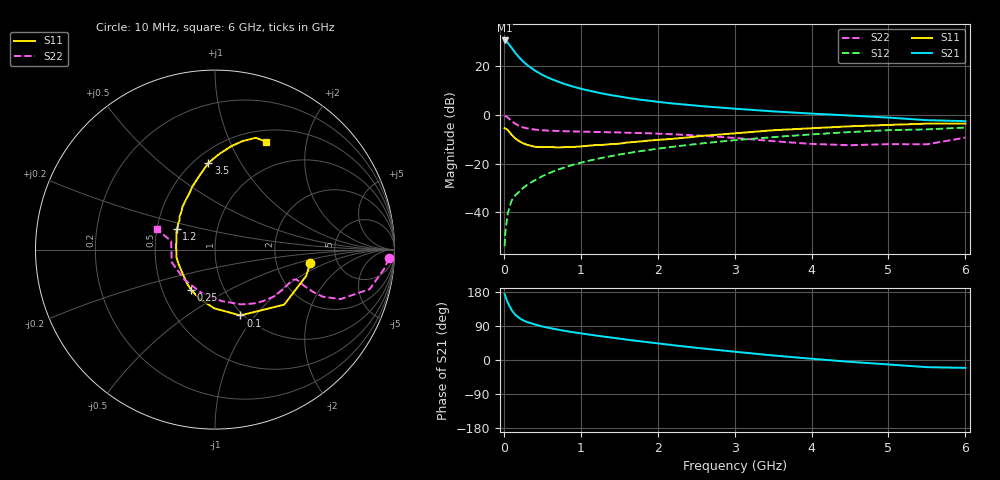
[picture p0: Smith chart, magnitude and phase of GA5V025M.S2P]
! Infineon Technologies  Discrete & RF Semiconductors
! BF775
! Si NPN RF Bipolar Junction Transistor in SOT23
! VCE = 5 V  IC = 25 mA
! Common Emitter S-Parameters:  May  1996
# GHz  S  MA  R  50
!  f  S11  S21  S12  S22
! GHz  MAG  ANG  MAG  ANG  MAG  ANG  MAG  ANG
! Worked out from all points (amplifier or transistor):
!   36 points, 10 MHz to 6 GHz, reference 50 ohm
!   highest |S21| = 30.7 dB at 10 MHz (marker M1)
!   |S21| within 3 dB of that: start of sweep to 100.5 MHz
!   unconditionally stable (mu >= 1): 352.7 MHz to 2.789 GHz
!   at 250 MHz: K = 0.91, MSG = 26.1 dB, |S12| = -30.1 dB
!   at 1.4 GHz: K = 1.11, MAG = 10.5 dB, |S12| = -16.9 dB
!   at 6 GHz: K = 0.93, MSG = 1.3 dB, |S12| = -5.2 dB
!   S11 on the Smith chart (normalised r, x): 10 MHz: 3.15, -0.68; 100 MHz: 0.97, -0.84; 250 MHz: 0.70, -0.34; 1.2 GHz: 0.63, +0.15; 3.5 GHz: 0.58, +0.74; 6 GHz: 0.64, +1.38
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0.01  0.5361 -8.2  34.09 173.7  0.002 89.1  0.9692 -2.9
0.02  0.5286 -16.2  33.6 167.6  0.0039 79.8  0.951 -6.2
0.05  0.4926 -38.5  30.77 151.7  0.0094 74.7  0.8898 -14.3
0.1  0.3932 -68.9  24.2 132.0  0.0172 69.1  0.7525 -21.5
0.15  0.3277 -90.5  18.89 119.0  0.0225 66.7  0.6557 -23.6
0.2  0.2886 -106.9  15.24 110.8  0.0264 67.3  0.5943 -23.3
0.25  0.2616 -120.3  12.61 104.8  0.0313 68.2  0.5559 -22.6
0.3  0.2443 -129.8  10.76 100.4  0.0364 69.5  0.5315 -22.0
0.4  0.222 -146.6  8.281 94.0  0.0452 71.0  0.501 -20.7
0.5  0.2182 -159.8  6.676 88.4  0.055 71.8  0.4844 -20.3
0.6  0.219 -169.0  5.633 84.2  0.0647 72.0  0.4756 -20.5
0.7  0.2155 -178.9  4.872 80.2  0.0746 71.8  0.4682 -21.0
0.8  0.2178 175.5  4.286 76.7  0.0845 71.0  0.4631 -21.9
0.9  0.2193 169.2  3.829 73.3  0.0943 71.1  0.4579 -22.7
1.1  0.2328 157.3  3.184 67.4  0.1138 69.8  0.451 -25.4
1.2  0.2412 152.0  2.941 64.4  0.1237 69.1  0.447 -26.5
1.6  0.271 136.6  2.256 53.7  0.1632 65.3  0.431 -33.0
2.2  0.3241 119.6  1.719 39.1  0.2223 59.5  0.4009 -44.4
3.5  0.485 94.3  1.186 12.0  0.3503 43.9  0.2895 -82.5
4.5  0.5846 80.9  0.973 -4.8  0.4456 30.4  0.2389 -135.2
5.5  0.6632 69.9  0.781 -18.9  0.5054 14.8  0.249 169.0
6  0.6647 64.6  0.746 -20.8  0.5513 10.4  0.3425 160.7
